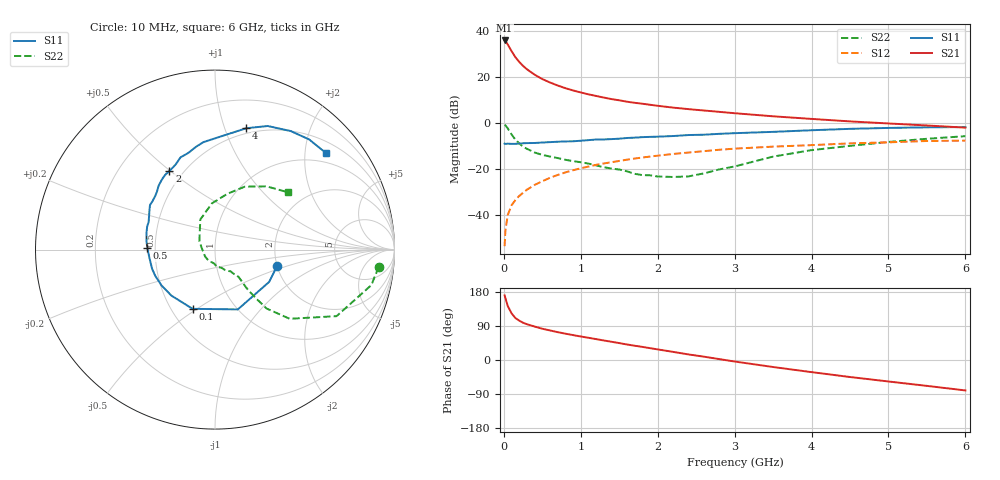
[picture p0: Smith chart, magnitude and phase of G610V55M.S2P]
! SIEMENS Small Signal Semiconductors
! BFG193
! Si NPN RF Bipolar Junction Transistor in SOT223
! VCE = 10 V  IC = 55 mA
! Common Emitter S-Parameters:  August  1996
# GHz  S  MA  R  50
!  f  S11  S21  S12  S22
! GHz  MAG  ANG  MAG  ANG  MAG  ANG  MAG  ANG
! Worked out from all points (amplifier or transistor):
!   36 points, 10 MHz to 6 GHz, reference 50 ohm
!   highest |S21| = 35.9 dB at 10 MHz (marker M1)
!   |S21| within 3 dB of that: start of sweep to 72.06 MHz
!   unconditionally stable (mu >= 1): 469.3 MHz to 2.448 GHz
!   at 250 MHz: K = 0.90, MSG = 27.6 dB, |S12| = -30.3 dB
!   at 1.4 GHz: K = 1.04, MAG = 12.5 dB, |S12| = -17.0 dB
!   at 6 GHz: K = 0.89, MSG = 2.8 dB, |S12| = -7.6 dB
!   S11 on the Smith chart (normalised r, x): 10 MHz: 1.99, -0.43; 100 MHz: 0.64, -0.48; 500 MHz: 0.45, +0.01; 2 GHz: 0.42, +0.50; 4 GHz: 0.45, +1.19; 6 GHz: 0.75, +2.47
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0.01  0.3575 -15.2  62.64 170.6  0.0021 86.7  0.9171 -6.1
0.02  0.3513 -30.9  60.68 163.5  0.0045 76.7  0.8932 -12.8
0.05  0.3567 -69.1  51.43 142.9  0.0099 70.7  0.7722 -28.7
0.1  0.3528 -110.7  36.76 123.2  0.0163 65.9  0.5673 -42.8
0.15  0.3532 -133.5  27.11 110.8  0.0211 64.8  0.4361 -48.8
0.2  0.3587 -146.3  21.41 103.9  0.026 66.7  0.3614 -49.8
0.25  0.3636 -156.1  17.5 98.3  0.0304 66.8  0.3064 -50.5
0.3  0.3664 -163.1  14.81 94.4  0.0355 68.0  0.2755 -50.6
0.4  0.3688 -173.7  11.29 88.3  0.0452 68.3  0.2292 -49.8
0.5  0.3773 178.5  9.068 82.5  0.0543 67.6  0.2031 -49.2
0.6  0.385 172.7  7.625 78.0  0.0645 66.8  0.1872 -50.0
0.8  0.3988 161.5  5.737 69.5  0.0844 63.8  0.159 -53.4
1.1  0.4251 149.3  4.215 58.6  0.1131 59.1  0.1312 -62.7
1.6  0.4735 131.7  2.916 41.0  0.1596 48.3  0.0893 -87.1
2  0.5059 120.1  2.375 28.0  0.1954 39.5  0.0688 -127.8
2.2  0.5221 114.9  2.169 21.4  0.2127 34.9  0.0672 -146.0
2.8  0.5832 100.3  1.753 2.4  0.2626 21.1  0.0981 152.1
3.5  0.6437 84.3  1.403 -18.5  0.3073 4.0  0.1865 116.0
4  0.6979 75.6  1.231 -32.0  0.3311 -5.7  0.2579 93.9
4.5  0.7486 66.9  1.087 -44.9  0.3617 -15.8  0.3191 77.4
5.5  0.8073 49.5  0.886 -68.3  0.4077 -39.0  0.4552 50.7
6  0.8193 41.1  0.795 -80.3  0.4147 -52.4  0.5184 37.9
